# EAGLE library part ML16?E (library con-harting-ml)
HARTING
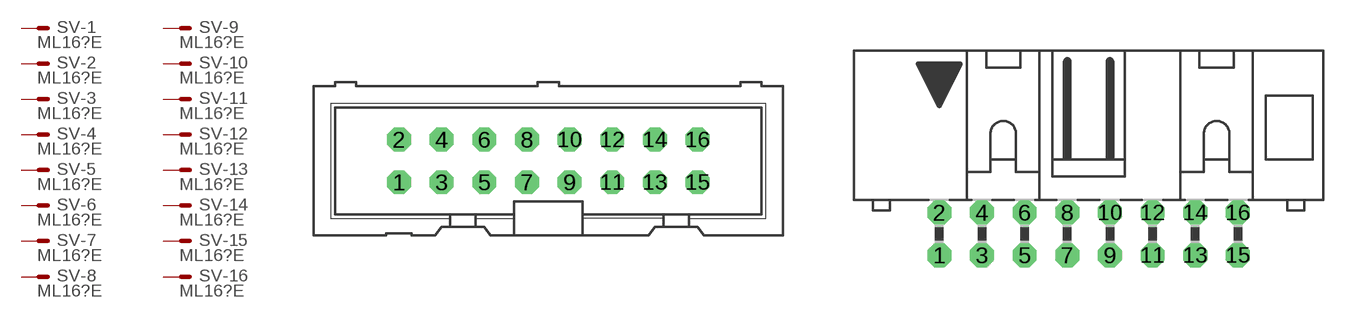
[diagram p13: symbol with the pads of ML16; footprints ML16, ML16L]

Designator prefix SV; gates -1=M -2=M -3=M -4=M -5=M -6=M -7=M -8=M -9=M -10=M -11=M -12=M -13=M -14=M -15=M -16=M

## ML16E (OC_FARNELL: unknown; OC_NEWARK: unknown)  [ML16]
1  -1:S  pas
2  -2:S  pas
3  -3:S  pas
4  -4:S  pas
5  -5:S  pas
6  -6:S  pas
7  -7:S  pas
8  -8:S  pas
9  -9:S  pas
10  -10:S  pas
11  -11:S  pas
12  -12:S  pas
13  -13:S  pas
14  -14:S  pas
15  -15:S  pas
16  -16:S  pas

## ML16LE (OC_FARNELL: unknown; OC_NEWARK: unknown)  [ML16L]
Pads as for ML16

## ML163ME (OC_FARNELL: unknown; OC_NEWARK: unknown)  [3M_16]
Pads as for ML16

## ML163MLE (OC_FARNELL: unknown; OC_NEWARK: unknown)  [3M_16L]
Pads as for ML16

## Footprint ML16 (pad centres in mm)
HARTING
drill 0.914 octagon: 1 -8.89,-1.27; 2 -8.89,1.27; 3 -6.35,-1.27; 4 -6.35,1.27; 5 -3.81,-1.27; 6 -3.81,1.27; 7 -1.27,-1.27; 8 -1.27,1.27; 9 1.27,-1.27; 10 1.27,1.27; 11 3.81,-1.27; 12 3.81,1.27; 13 6.35,-1.27; 14 6.35,1.27; 15 8.89,-1.27; 16 8.89,1.27

## Footprint ML16L (pad centres in mm)
HARTING
drill 0.914 octagon: 1 -8.89,-1.27; 2 -8.89,1.27; 3 -6.35,-1.27; 4 -6.35,1.27; 5 -3.81,-1.27; 6 -3.81,1.27; 7 -1.27,-1.27; 8 -1.27,1.27; 9 1.27,-1.27; 10 1.27,1.27; 11 3.81,-1.27; 12 3.81,1.27; 13 6.35,-1.27; 14 6.35,1.27; 15 8.89,-1.27; 16 8.89,1.27

## Footprint 3M_16 (pad centres in mm)
3M
drill 0.813 square: 1 -8.89,-1.27; 2 -8.89,1.27; 3 -6.35,-1.27; 4 -6.35,1.27; 5 -3.81,-1.27; 6 -3.81,1.27; 7 -1.27,-1.27; 8 -1.27,1.27; 9 1.27,-1.27; 10 1.27,1.27; 11 3.81,-1.27; 12 3.81,1.27; 13 6.35,-1.27; 14 6.35,1.27; 15 8.89,-1.27; 16 8.89,1.27

## Footprint 3M_16L (pad centres in mm)
3M
drill 0.813 square: 1 -8.89,-5.08; 2 -8.89,-2.54; 3 -6.35,-5.08; 4 -6.35,-2.54; 5 -3.81,-5.08; 6 -3.81,-2.54; 7 -1.27,-5.08; 8 -1.27,-2.54; 9 1.27,-5.08; 10 1.27,-2.54; 11 3.81,-5.08; 12 3.81,-2.54; 13 6.35,-5.08; 14 6.35,-2.54; 15 8.89,-5.08; 16 8.89,-2.54
hole 2.54 at -14.808,-3.277
hole 2.54 at 14.808,-3.277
